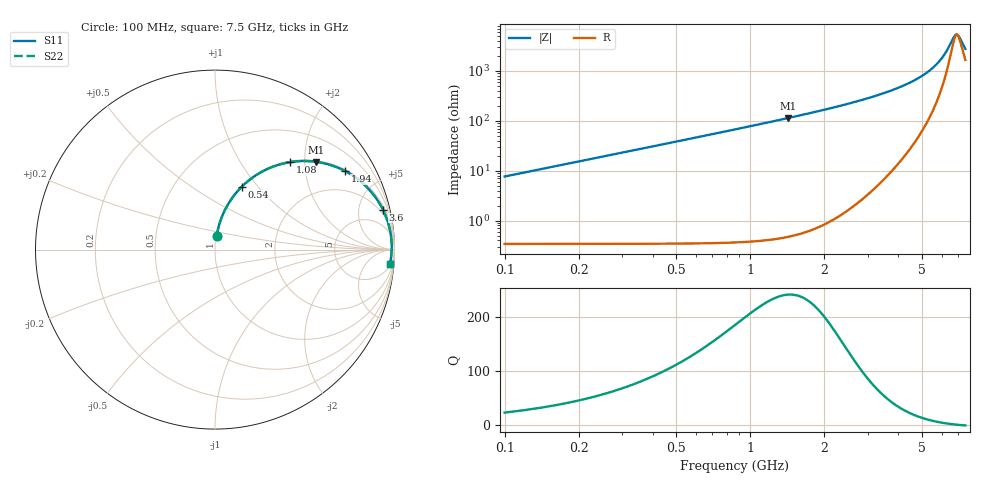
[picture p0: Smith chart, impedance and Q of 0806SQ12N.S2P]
! Coilcraft 0806SQ-12N Air Core Inductor
! 06 March 2008
# MHZ S MA R 50
!Freq  MagS11  AngS11  MagS21  AngS21  MagS12  AngS12  MagS22  AngS22
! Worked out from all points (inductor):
!   371 points, 100 MHz to 7.5 GHz, reference 50 ohm
!   read as one part in series: L = 12.2 nH near 120 MHz
!   highest Q = 241 at 1.42 GHz (marker M1), where L = 12.7 nH
!   self-resonance near 6.939 GHz
!   S11 on the Smith chart (normalised r, x): 100 MHz: 1.01, +0.15; 540 MHz: 1.01, +0.83; 1.08 GHz: 1.02, +1.70; 1.94 GHz: 1.06, +3.28; 3.6 GHz: 1.40, +8.29; 7.5 GHz: 6, -23
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100  0.07572 83.1  0.9937 -4.4  0.9937 -4.4  0.07573 83.1
160  0.1206 81.4  0.9893 -7.0  0.9893 -7.0  0.1206 81.4
200  0.1501 80.0  0.9853 -8.7  0.9853 -8.7  0.1502 80.0
260  0.1938 77.7  0.9777 -11.3  0.9777 -11.3  0.1938 77.7
380  0.2777 73.1  0.9574 -16.3  0.9574 -16.3  0.2778 73.1
540  0.381 66.9  0.9214 -22.6  0.9214 -22.6  0.3811 66.9
780  0.514 58.4  0.8547 -31.2  0.8547 -31.2  0.514 58.4
1080  0.643 49.3  0.7629 -40.4  0.7629 -40.4  0.643 49.3
1340  0.7259 42.7  0.6847 -47.1  0.6847 -47.1  0.7259 42.7
1420  0.747 40.9  0.6617 -48.9  0.6617 -48.9  0.747 40.9
1940  0.8467 31.1  0.5279 -58.6  0.5279 -58.6  0.8468 31.1
2580  0.9134 22.6  0.3998 -67.0  0.3998 -67.0  0.9134 22.6
3600  0.9616 13.4  0.2552 -75.4  0.2552 -75.4  0.9616 13.4
3800  0.9667 12.0  0.2328 -76.6  0.2328 -76.6  0.9668 12.0
5040  0.9829 4.9  0.1202 -80.4  0.1202 -80.4  0.9829 4.9
5740  0.9848 1.8  0.07138 -78.0  0.07138 -78.0  0.9848 1.8
6020  0.9846 0.6  0.05421 -74.5  0.05421 -74.5  0.9847 0.6
6280  0.9842 -0.4  0.03966 -68.0  0.03966 -68.0  0.9842 -0.4
6720  0.9827 -2.0  0.02082 -36.2  0.02082 -36.2  0.9827 -2.0
6900  0.9819 -2.6  0.01822 -9.1  0.01822 -9.1  0.9819 -2.6
7060  0.981 -3.2  0.01994 15.3  0.01994 15.3  0.9811 -3.2
7500  0.9784 -4.6  0.0353 48.4  0.0353 48.4  0.9784 -4.6
